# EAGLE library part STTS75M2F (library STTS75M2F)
STTS75M2F, 12bit Temperature Sensor +/-3C Serial-I2C 2.7 to 5.5V 8-Pin SOIC Source: Datasheet
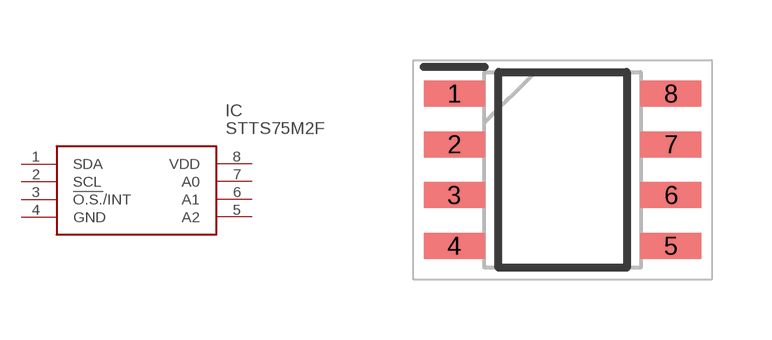
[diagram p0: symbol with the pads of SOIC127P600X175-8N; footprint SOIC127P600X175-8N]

Designator prefix IC

## STTS75M2F (Description: STTS75M2F, 12bit Temperature Sensor +/-3C Serial-I2C 2.7 to 5.5V 8-Pin SOIC; Height: 1.75mm; Manufacturer_Name: STMicroelectronics; Manufacturer_Part_Number: STTS75M2F; Mouser_Part_Number: 511-STTS75M2F; Mouser_Price-Stock: https://www.mouser.com/Search/Refine.aspx?Keyword=511-STTS75M2F)  [SOIC127P600X175-8N]
1  SDA
2  SCL
3  !O.S.!/INT
4  GND
5  A2
6  A1
7  A0
8  VDD

## Footprint SOIC127P600X175-8N (pad centres in mm)
SO 8_
smd 1.525 x 0.65: 1 -2.712,1.905; 2 -2.712,0.635; 3 -2.712,-0.635; 4 -2.712,-1.905; 5 2.712,-1.905; 6 2.712,-0.635; 7 2.712,0.635; 8 2.712,1.905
